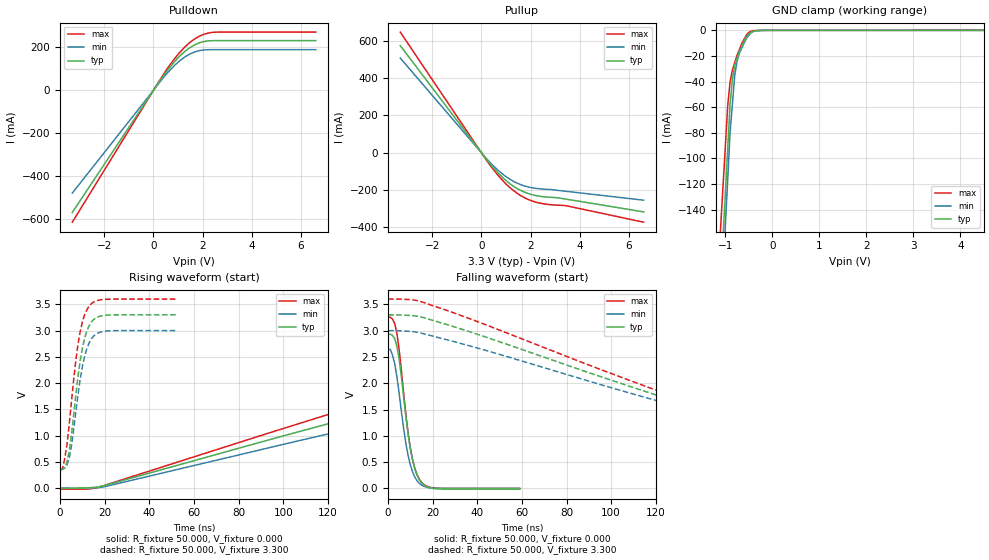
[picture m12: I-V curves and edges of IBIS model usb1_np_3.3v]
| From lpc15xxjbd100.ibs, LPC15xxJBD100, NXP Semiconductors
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[Model]   usb1_np_3.3v
Model_type I/O
Vinl=9.900E-01
Vinh=2.310E+00
Vref=0.000E+00
Rref=1.000E+06
Cref=0.000E+00
Vmeas=1.650E+00
C_comp   2.000E-12   2.000E-12   2.000E-12
[Voltage Range]   3.300E+00   3.000E+00   3.600E+00
[POWER Clamp Reference]   3.300E+00   3.000E+00   3.600E+00
[GND Clamp Reference]   0.000E+00   0.000E+00   0.000E+00
[Pullup Reference]   3.300E+00   3.000E+00   3.600E+00
[Pulldown Reference]   0.000E+00   0.000E+00   0.000E+00
[Temperature Range]   25   85   -40
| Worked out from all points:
|   slope of the pulldown table from 0 to 0.495 V, typ, clamps not added: 6.06 ohm
|   slope of the pullup table from 0 to 0.495 V, typ, clamps not added: 6.04 ohm
|   GND clamp passes 1 mA (typ) near -0.43 V on its own axis
|   rising waveform, R_fixture 50.000, V_fixture 0.000: 20-80 % time 164ns typ, 173ns min, 155ns max; typ from 0 V to 2.96 V
|   falling waveform, R_fixture 50.000, V_fixture 0.000: 20-80 % time 5.51ns typ, 5.54ns min, 5.45ns max; typ from 2.93 V to -0.014 V
|   rising waveform, R_fixture 50.000, V_fixture 3.300: 20-80 % time 5.37ns typ, 5.43ns min, 5.35ns max; typ from 0.352 V to 3.3 V
|   falling waveform, R_fixture 50.000, V_fixture 3.300: 20-80 % time 127ns typ, 132ns min, 123ns max; typ from 3.3 V to 0.352 V
[GND Clamp]
-3.3V     -1.714A    -1.818A    -1.535A
-950mV    -92.32mA   -116.3mA   -58.79mA
-900mV    -57.82mA   -80.06mA   -40.13mA
-850mV    -38.01mA   -57.45mA   -30.95mA
-800mV    -27.38mA   -34.83mA   -25.11mA
-750mV    -21.67mA   -23.95mA   -19.28mA
-700mV    -15.97mA   -17.62mA   -14.76mA
-550mV    -4.988mA   -6.167mA   -3.507mA
-450mV    -1.299mA   -1.865mA   -600.8uA
-350mV    -373.3uA   -390uA     -110.4uA
-125mV    -16.52uA   -11.27uA   -3.965uA
6.6V      10.68uA    9.931uA    4.357uA
[Power Clamp]
-3.3V     0A         0A         0A
0V        0A         0A         0A
3.3V      0A         0A         0A
6.6V      0A         0A         0A
[Pullup]
-3.3V     573.9mA    507.4mA    646.2mA
260mV     -45.14mA   -39.12mA   -50.35mA
720mV     -114.4mA   -98.69mA   -128mA
1.02V     -151.1mA   -130mA     -170.2mA
1.28V     -177.4mA   -151.7mA   -200.2mA
1.8V      -213.8mA   -180.2mA   -244.2mA
2.34V     -232.8mA   -193.1mA   -269.2mA
2.74V     -238.6mA   -196.9mA   -277.9mA
3.44V     -248.8mA   -206.9mA   -284.2mA
6.6V      -317.3mA   -254.6mA   -372.5mA
[Pulldown]
-3.3V     -569.7mA   -479mA     -615.1mA
420mV     69.92mA    61.22mA    76.39mA
1V        151.6mA    131.1mA    167.7mA
1.48V     198.8mA    169.2mA    223.1mA
1.94V     224mA      186.5mA    256.1mA
2.44V     231.7mA    189.6mA    270.6mA
6.6V      231.7mA    189.6mA    271.6mA
[Rising Waveform]
R_fixture = 50.000
V_fixture = 0.000
V_fixture_min = 0.000
V_fixture_max = 0.000
|  time   V(typ)   V(min)   V(max)
0s        82.46uV    62.66uV    -17.02mV
17ns      24.36mV    10.81mV    15.03mV
112ns     1.134V     953.9mV    1.296V
168ns     1.756V     1.488V     2.007V
223ns     2.308V     1.964V     2.631V
254ns     2.558V     2.194V     2.889V
293ns     2.746V     2.391V     3.061V
352ns     2.872V     2.538V     3.161V
417ns     2.924V     2.605V     3.203V
513ns     2.955V     2.643V     3.228V
[Falling Waveform]
R_fixture = 50.000
V_fixture = 0.000
V_fixture_min = 0.000
V_fixture_max = 0.000
|  time   V(typ)   V(min)   V(max)
0s        2.931V     2.643V     3.255V
2ns       2.91V      2.533V     3.221V
4ns       2.698V     2.112V     2.936V
5ns       2.449V     1.795V     2.627V
8ns       1.359V     852.2mV    1.398V
10ns      753.5mV    446.1mV    762.7mV
12ns      374.8mV    215mV      378.2mV
15ns      108.7mV    63.37mV    116mV
22ns      -8.347mV   2.59mV     5.02mV
59ns      -13.87mV   62.66uV    18.21uV
[Rising Waveform]
R_fixture = 50.000
V_fixture = 3.300
V_fixture_min = 3.000
V_fixture_max = 3.600
|  time   V(typ)   V(min)   V(max)
0s        351.9mV    365.5mV    361.3mV
1ns       353.9mV    365.5mV    360.4mV
2ns       389.9mV    379.4mV    553.4mV
4ns       689.2mV    561.4mV    1.191V
6ns       1.375V     1.095V     2.047V
8ns       2.128V     1.78V      2.74V
10ns      2.674V     2.324V     3.17V
13ns      3.093V     2.766V     3.467V
20ns      3.29V      2.988V     3.594V
52ns      3.3V       3V         3.6V
[Falling Waveform]
R_fixture = 50.000
V_fixture = 3.300
V_fixture_min = 3.000
V_fixture_max = 3.600
|  time   V(typ)   V(min)   V(max)
0s        3.3V       3V         3.6V
12ns      3.281V     2.977V     3.579V
24ns      3.145V     2.852V     3.419V
144ns     1.448V     1.388V     1.496V
184ns     925mV      936.1mV    906.2mV
206ns     672.8mV    712.6mV    636.6mV
225ns     529mV      571.6mV    504.3mV
249ns     437.8mV    471.3mV    427.9mV
285ns     381.7mV    403.2mV    384.3mV
339ns     351.9mV    365.5mV    361.3mV
[Ramp]
dV/dt_r   1.7668E+00/1.6350E-07   1.5807E+00/1.7195E-07   1.9467E+00/1.5631E-07
dV/dt_f   1.7689E+00/1.2734E-07   1.5807E+00/1.3210E-07   1.9432E+00/1.2325E-07
R_load = 50
